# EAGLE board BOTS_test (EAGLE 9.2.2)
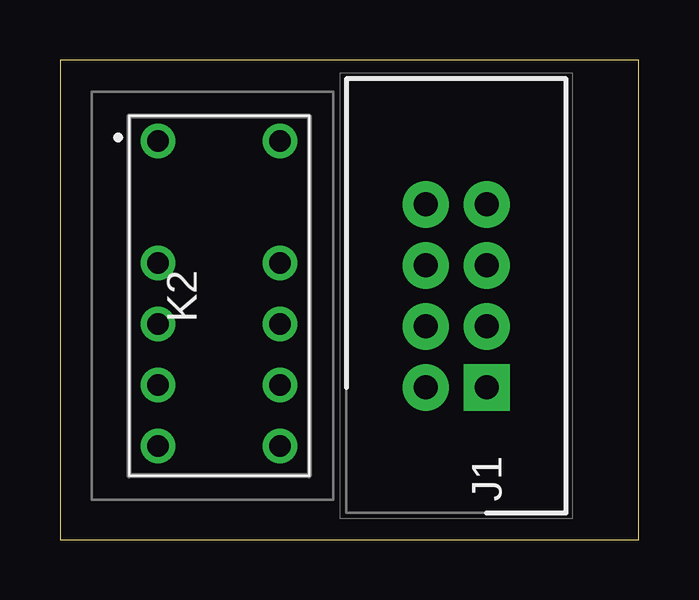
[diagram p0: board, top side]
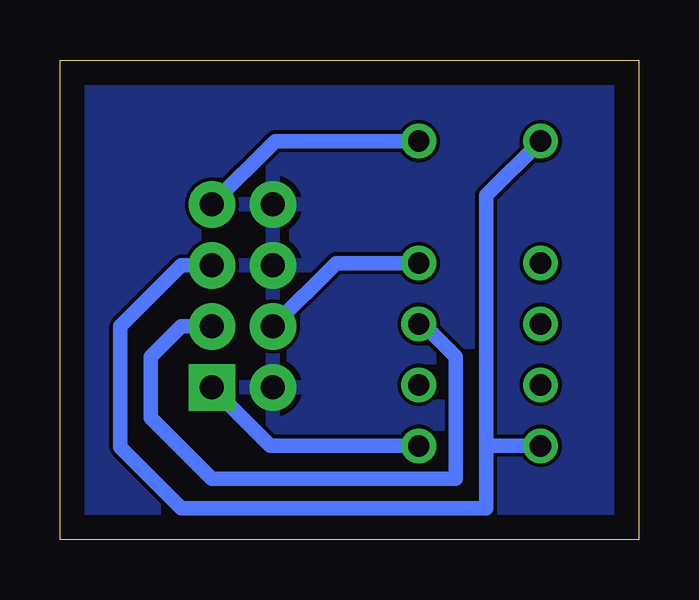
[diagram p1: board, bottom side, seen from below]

Size 24.11 x 19.99 mm. Coordinates in mm from the lower left corner, seen from the top.
Outline: 0,0 24.11,0 24.11,19.99 0,19.99 0,0
Copper layers (1*16): Top 0.035mm / dielectric 1.5mm / Bottom 0.035mm
Design rules "default": minimum track width 6mil, minimum drill 0.35mm, track to track 6mil, track to pad 6mil, pad to pad 6mil, via to via 6mil, smd to smd 6mil, copper to edge 40mil, drill to drill 6mil, minimum pad ring 10mil, minimum via ring 8mil, stop-mask expansion 4mil, vias tented up to drill 0mil, thermal gap 10mil

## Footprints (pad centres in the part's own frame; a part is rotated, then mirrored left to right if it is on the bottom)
HDRV8W64P254_2X4_1778X895X915P = drill 1 pad 1.93 square: 1 0,0 | drill 1 pad 1.93: 2 0,2.54; 3 2.54,0; 4 2.54,2.54; 5 5.08,0; 6 5.08,2.54; 7 7.62,0; 8 7.62,2.54
EC212TNU = drill 0.89 pad 1.446: 1 -6.45,-2.265; 3 -1.37,-2.265; 4 1.17,-2.265; 5 3.71,-2.265; 6 6.25,-2.265; 7 6.25,2.815; 8 3.71,2.815; 9 1.17,2.815; 10 -1.37,2.815; 12 -6.45,2.815

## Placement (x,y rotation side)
J1  ASS + BOTS  [HDRV8W64P254_2X4_1778X895X915P]  17.78,6.35 90 top
K2  EC2-12TNU  [EC212TNU]  6.35,10.16 270 top

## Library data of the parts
J1 = T821108A1S100CEU; DESCRIPTION: HEADER, VERTICAL, 2.54MM, 8WAY Amphenol T821 Series, 2.54mm Pitch 8 Way 2 Row Straight PCB Header, Solder Termination, 3A; HEIGHT: 9.15mm; MANUFACTURER_NAME: Amphenol; MANUFACTURER_PART_NUMBER: T821108A1S100CEU; RS_PART_NUMBER: 1702738
K2 = SamacSys_Parts; DESCRIPTION: DPDT Through Hole Latching Relay, 2 A, 12V dc; HEIGHT: 9mm; MANUFACTURER_NAME: Kemet; MANUFACTURER_PART_NUMBER: EC2-12TNU; MOUSER_PART_NUMBER: 80-EC2-12TNU

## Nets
12V: J1.5 K2.1 K2.6
ASS1: J1.4 K2.10
GND: J1.2 J1.6 J1.8
N$1: J1.1 K2.7
N$2: J1.7 K2.12
N$3: J1.3 K2.9

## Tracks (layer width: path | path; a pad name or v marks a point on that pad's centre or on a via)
12V
  Bottom 0.61: J1.5 19.05,11.43 21.59,8.89 21.59,3.86 19.05,1.32 6.35,1.32 6.35,3.81 | K2.6 6.25,3.91 6.35,3.81 | 6.35,3.81 6.35,14.35 K2.1
ASS1
  Bottom 0.61: K2.10 12.6,11.53 J1.4
GND
  pour Bottom: 0,0 24.13,0 24.13,20.32 0,20.32
N$1
  Bottom 0.61: K2.7 15.34,3.91 J1.1
N$2
  Bottom 0.61: K2.12 15.14,16.61 J1.7
N$3
  Bottom 0.61: K2.9 8.99,8.99 7.62,7.62 7.62,2.54 17.78,2.54 20.32,5.08 20.32,7.62 19.05,8.89 J1.3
